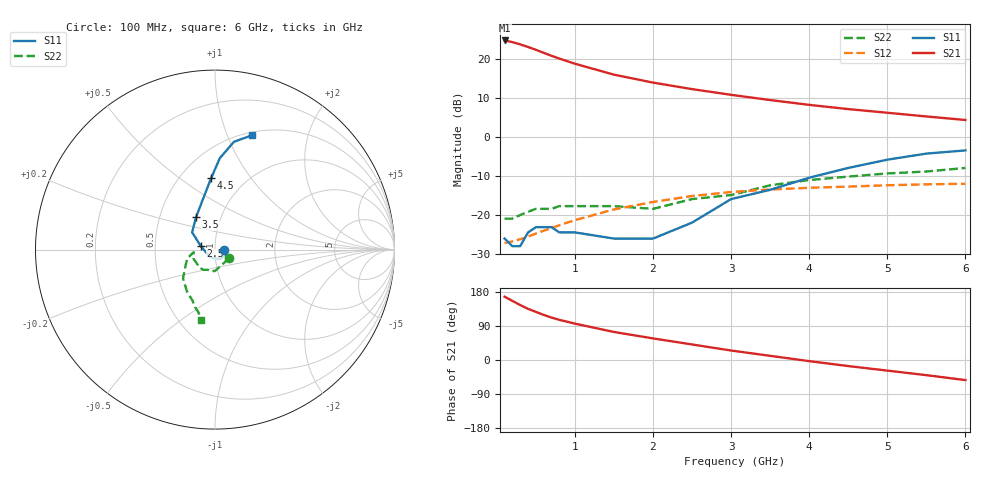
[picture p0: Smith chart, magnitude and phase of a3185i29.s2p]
!  MSA-3185 S AND NOISE PARAMETERS
!  Id = 29 mA  LAST UPDATED 07-01-94
# ghz s ma r 50
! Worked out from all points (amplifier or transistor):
!   20 points, 100 MHz to 6 GHz, reference 50 ohm
!   highest |S21| = 24.6 dB at 100 MHz (marker M1)
!   |S21| within 3 dB of that: start of sweep to 579.9 MHz
!   unconditionally stable (mu >= 1): start of sweep to 3.389 GHz
!   at 400 MHz: K = 1.03, MAG = 23.1 dB, |S12| = -25.5 dB
!   at 1.5 GHz: K = 1.03, MAG = 16.2 dB, |S12| = -18.6 dB
!   at 6 GHz: K = 0.59, MSG = 8.2 dB, |S12| = -12.0 dB
!   S11 on the Smith chart (normalised r, x): 100 MHz: 1.11, -0.01; 2.5 GHz: 0.85, +0.03; 3.5 GHz: 0.76, +0.29; 4.5 GHz: 0.70, +0.66; 6 GHz: 0.53, +1.23
0.1  0.05 -3.0  17.04 167.0  0.044 8.0  0.09 -32.0
0.2  0.04 -13.0  16.22 156.0  0.046 16.0  0.09 -57.0
0.3  0.04 -22.0  15.18 145.0  0.049 22.0  0.1 -76.0
0.4  0.06 -25.0  14.07 135.0  0.053 27.0  0.11 -84.0
0.5  0.07 -27.0  12.95 127.0  0.058 31.0  0.12 -91.0
0.6  0.07 -31.0  11.85 119.0  0.063 34.0  0.12 -102.0
0.7  0.07 -33.0  10.85 112.0  0.068 36.0  0.12 -110.0
0.8  0.06 -41.0  10.01 106.0  0.074 38.0  0.13 -120.0
0.9  0.06 -45.0  9.27 101.0  0.08 39.0  0.13 -126.0
1  0.06 -57.0  8.59 96.0  0.086 40.0  0.13 -134.0
1.5  0.05 -89.0  6.23 74.0  0.118 38.0  0.13 -157.0
2  0.05 -122.0  4.93 57.0  0.147 33.0  0.12 -173.0
2.5  0.08 167.0  4.07 41.0  0.175 26.0  0.16 -163.0
3  0.16 143.0  3.44 25.0  0.197 17.0  0.18 -154.0
3.5  0.21 120.0  2.95 11.0  0.212 9.0  0.24 -138.0
4  0.3 102.0  2.56 -3.0  0.223 2.0  0.28 -124.0
4.5  0.4 93.0  2.26 -16.0  0.231 -5.0  0.31 -114.0
5  0.51 87.0  2.03 -28.0  0.24 -11.0  0.34 -109.0
5.5  0.61 80.0  1.82 -40.0  0.247 -17.0  0.36 -105.0
6  0.67 72.0  1.64 -53.0  0.251 -23.0  0.4 -101.0
